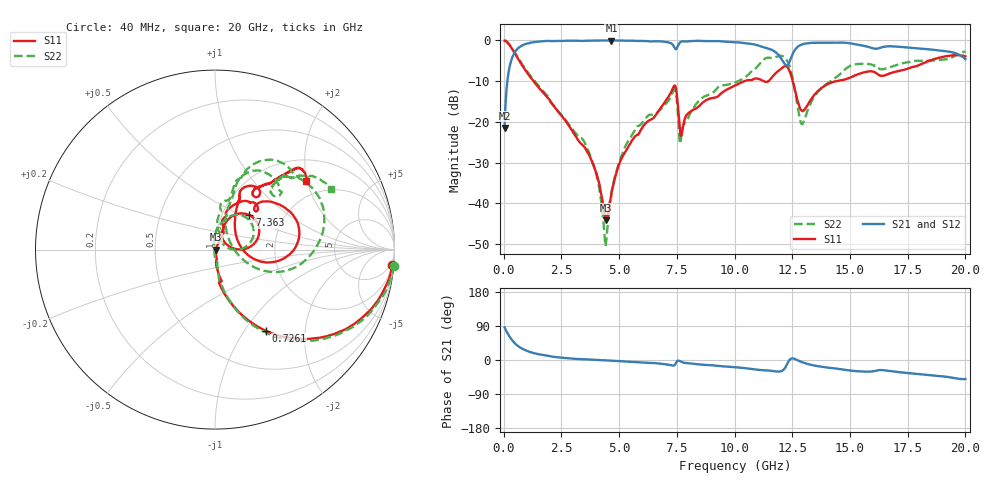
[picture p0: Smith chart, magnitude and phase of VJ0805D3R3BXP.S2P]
! VJ0805D3R3BXP
! DATE 10/29/2021  11:45
! CAPACITORS MOUNTED IN SERIES ON 25 MIL THICK MICROSTRIP SUBSTRATE
# GHz  S  MA  R  50.00
!  FREQ  S11M  S11A  S21M  S21A  S12M  S12A  S22M  S22A
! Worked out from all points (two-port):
!   1601 points, 40 MHz to 20 GHz, reference 50 ohm
!   highest |S21| = -0.02 dB at 4.668 GHz (marker M1); lowest = -21.5 dB at 40 MHz (marker M2)
!   |S21| within 3 dB of the highest: 469 MHz to 11.81 GHz (11.34 GHz wide, 185 % of centre); 12.54 GHz to 19.49 GHz (6.953 GHz wide, 43.4 % of centre)
!   lowest |S11| = -44.2 dB at 4.444 GHz (marker M3), VSWR 1.01, Z = 50.6 - j0.0999 ohm
!   |S11| at or under -10 dB: 1.289 GHz to 10.43 GHz (9.141 GHz wide, 156 % of centre); 11.26 GHz to 11.47 GHz (204.9 MHz wide, 1.8 % of centre); 12.52 GHz to 14.4 GHz (1.881 GHz wide, 14 % of centre)
!   |S22| runs from -50.5 to 0.0 dB; largest |S21 - S12| = 0.012
!   S11 on the Smith chart (normalised r, x): 40 MHz: 2, -23; 726.1 MHz: 0.99, -1.26; 7.363 GHz: 1.34, +0.56; 20 GHz: 1.53, +1.97
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0.04  0.9923 -4.9  0.08404 86.1  0.0817 84.2  0.9994 -5.1
0.2895  0.8517 -31.4  0.5207 58.8  0.5193 58.6  0.8576 -31.5
0.726125  0.5341 -58.0  0.8452 32.5  0.8454 32.5  0.5473 -58.2
1.574425  0.2524 -77.7  0.9721 14.5  0.9718 14.4  0.2642 -76.2
3.370825  0.05346 -79.3  0.988 2.1  0.988 2.1  0.06277 -80.4
4.00705  0.02392 -76.7  0.9964 0.3  0.9969 0.2  0.02284 -96.7
4.443675  0.006201 -9.2  0.9967 -1.1  0.9967 -1.2  0.003468 155.8
4.668225  0.01351 50.6  0.9976 -1.8  0.9977 -2.0  0.01334 107.3
5.35435  0.04694 62.9  0.9933 -4.1  0.9932 -4.2  0.05535 96.0
6.70165  0.1348 68.8  0.9755 -9.1  0.9756 -9.2  0.1335 78.6
7.362825  0.2715 45.1  0.8541 -14.7  0.8537 -14.9  0.245 49.6
7.687175  0.06779 39.7  0.9667 -4.7  0.967 -4.8  0.06457 62.0
8.49805  0.159 75.8  0.9882 -11.9  0.9882 -12.0  0.1848 84.0
10.02  0.2794 65.3  0.9498 -19.0  0.9498 -19.1  0.3038 73.8
11.29245  0.3139 42.7  0.819 -27.1  0.8187 -27.2  0.5911 57.9
12.1158  0.472 25.5  0.5436 -26.0  0.5435 -26.2  0.6335 16.2
12.47757  0.3509 -10.7  0.6427 4.2  0.6428 3.9  0.3888 -18.4
12.88925  0.1387 12.6  0.8858 -4.8  0.8863 -5.0  0.09557 16.6
13.35083  0.196 55.2  0.9347 -13.2  0.9345 -13.4  0.1822 71.1
15.0599  0.3563 66.5  0.9173 -28.2  0.9171 -28.5  0.4941 62.9
16.68165  0.3892 56.8  0.8449 -28.9  0.8466 -29.6  0.4626 47.5
20  0.637 37.0  0.5905 -50.1  0.5885 -50.9  0.7307 27.6
